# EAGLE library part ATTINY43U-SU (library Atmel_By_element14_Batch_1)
8-bit Microcontroller with In-System Programmable Flash and Boost Converter
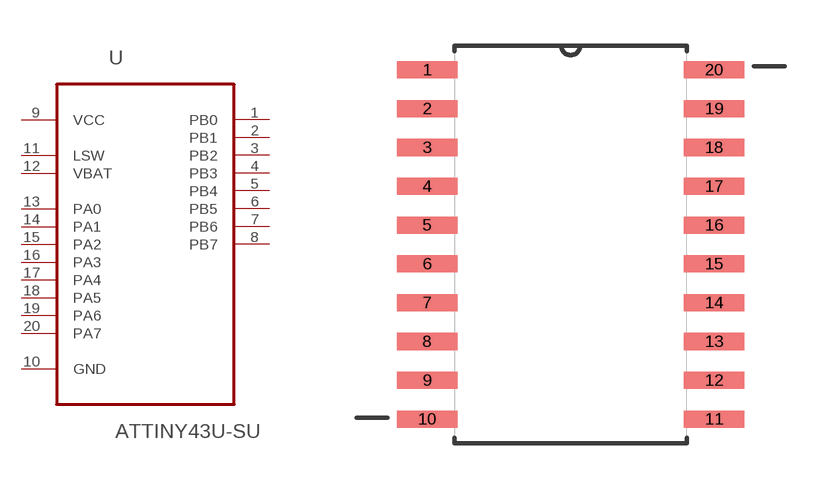
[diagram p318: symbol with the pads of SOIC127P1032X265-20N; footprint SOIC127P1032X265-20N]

Designator prefix U

## ATTINY43U-SU (MPN: ATTINY43U-SU; OC_FARNELL: 1841623; OC_NEWARK: 12T1338; PACKAGE: SOIC-20; SUPPLIER: Atmel)  [SOIC127P1032X265-20N]
1  PB0
2  PB1
3  PB2
4  PB3
5  PB4
6  PB5
7  PB6
8  PB7
9  VCC  pwr
10  GND  pas
11  LSW  pas
12  VBAT  pas
13  PA0
14  PA1
15  PA2
16  PA3
17  PA4
18  PA5
19  PA6
20  PA7

## Footprint SOIC127P1032X265-20N (pad centres in mm)
smd 1.981 x 0.559: 1 -4.699,5.715; 2 -4.699,4.445; 3 -4.699,3.175; 4 -4.699,1.905; 5 -4.699,0.635; 6 -4.699,-0.635; 7 -4.699,-1.905; 8 -4.699,-3.175; 9 -4.699,-4.445; 10 -4.699,-5.715; 11 4.699,-5.715; 12 4.699,-4.445; 13 4.699,-3.175; 14 4.699,-1.905; 15 4.699,-0.635; 16 4.699,0.635; 17 4.699,1.905; 18 4.699,3.175; 19 4.699,4.445; 20 4.699,5.715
